VAR_GLOBAL CONSTANT	
	
	cOversamples 	: UDINT 	:= 10;		// number of oversamples
	cFSample        : UDINT     := 10000;   // 1ms task with 10 oversamples = 10kHz
	
	// define FFT parameters, note that cFSample / cWindowLength must be such that numerical frequency resolution
	// is lower than fLowerFrequencyLimit resolution  =  10000/4000 = 2.5 Hz < 10 Hz 
	cFFTLength		: UDINT		:= 4096;	        // length of FFT
    cWindowLength   : UDINT     := 4000;            // 96 samples Zero padding
	cBufferLength	: UDINT		:= cWindowLength/2;	// buffer size due to 50% overlap
	
	// define frequency interval according to ISO 10816-3
	// e.g. 10 .. 1000 Hz for rotating speed over 600r/min
	cfLowerFrequencyLimit : UDINT := 10;   
	cfUpperFrequencyLimit : UDINT := 1000; 
	
	// Parameters for RMS calculation
	cOrderRMS        : UDINT := 2; // ISO 10816-3 requires velocity and displacement, if measured using accelerometer we need to integrate 2 times
	cChannels		 : UDINT := 2; // ISO 10816-3 says 2 orthogonal sensors per measurement location-> 2 channels
	cResult_Length   : UDINT := cOrderRMS+1; // nOrder+1
	
	// Classes according to ISO: machine type 1, stiff location, Class definitions
	cISOClassDef_Velocity  : ARRAY[1..3] OF LREAL := [2.3E-3, 4.5E-3, 7.1E-3];
	cISOClassDef_Displ     : ARRAY[1..3] OF LREAL := [29E-6, 57E-6, 90E-6];	
	
	// optional constants if real sensors are applied
	cGravitationalAcc : LREAL := 9.81;    // 1 g approx 9.81 m/s^2 -> physical constant
	cSensitivity      : LREAL := 0.01;    // [in Volts/g] depends on sensor used in application, e.g. 10 mV/g
	cMeasurementRange : LREAL := 5;       // +-5 Volts (EL3632)
	cResolution       : LREAL := 32768;   // 2^15 (15 bits resolution + 1 bit sign) (EL3632)
	cScale            : LREAL := cMeasurementRange*cGravitationalAcc/(cSensitivity*cResolution);
	
END_VAR
